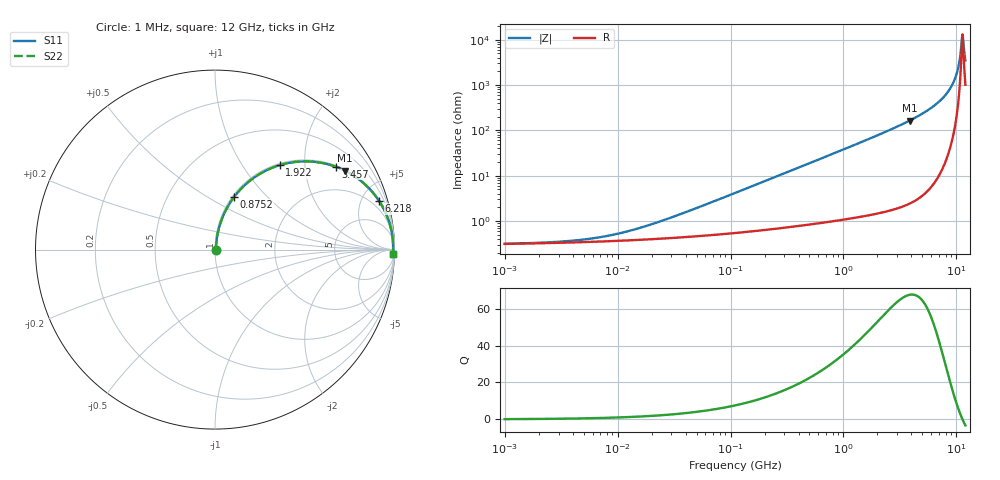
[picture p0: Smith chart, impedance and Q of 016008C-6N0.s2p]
# MHz S MA R 50
!Freq  MagS11  AngS11  MagS21  AngS21  MagS12  AngS12  MagS22  AngS22
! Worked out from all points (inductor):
!   801 points, 1 MHz to 12 GHz, reference 50 ohm
!   read as one part in series: L = 6 nH near 34.66 MHz
!   highest Q = 67.5 at 3.842 GHz (marker M1), where L = 6.78 nH
!   self-resonance near 11.18 GHz
!   S11 on the Smith chart (normalised r, x): 1 MHz: 1.01, +0.00; 875.2 MHz: 1.02, +0.66; 1.922 GHz: 1.03, +1.49; 3.457 GHz: 1.04, +2.87; 6.218 GHz: 1.13, +6.72; 12 GHz: 21, -66
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1  0.003158 6.8  0.9969 -0.0  0.9969 -0.0  0.003158 6.8
4.822396  0.003876 27.8  0.9966 -0.1  0.9966 -0.1  0.003876 27.8
10.34419  0.005348 46.4  0.9963 -0.2  0.9963 -0.2  0.005348 46.4
22.98406  0.009536 64.3  0.9959 -0.5  0.9959 -0.5  0.009536 64.3
110.8382  0.04188 80.1  0.9937 -2.4  0.9937 -2.4  0.04188 80.1
261.1649  0.09761 80.4  0.9885 -5.6  0.9885 -5.6  0.09761 80.4
528.267  0.1943 76.4  0.9727 -11.2  0.9727 -11.2  0.1943 76.4
875.2044  0.3123 70.0  0.9404 -18.2  0.9404 -18.2  0.3123 70.0
1304.592  0.442 62.4  0.8864 -26.2  0.8864 -26.2  0.442 62.4
1921.945  0.5926 52.6  0.7941 -36.3  0.7941 -36.3  0.5926 52.6
2517.778  0.7008 44.6  0.7017 -44.5  0.7017 -44.5  0.7008 44.6
3456.923  0.8152 34.5  0.567 -54.6  0.567 -54.6  0.8152 34.5
3842.205  0.8479 31.2  0.5178 -58.0  0.5178 -58.0  0.8479 31.2
6217.826  0.9535 16.5  0.2839 -72.4  0.2839 -72.4  0.9535 16.5
7863.54  0.9798 9.8  0.1709 -78.3  0.1709 -78.3  0.9798 9.8
9268.379  0.9896 5.3  0.09331 -80.9  0.09331 -80.9  0.9896 5.3
10181.12  0.9921 2.8  0.04961 -79.4  0.04961 -79.4  0.9921 2.8
10423.02  0.9924 2.2  0.03882 -77.6  0.03882 -77.6  0.9924 2.2
10924.19  0.9926 0.9  0.01789 -65.0  0.01789 -65.0  0.9926 0.9
11183.75  0.9925 0.3  0.009265 -35.4  0.009265 -35.4  0.9925 0.3
11584.69  0.992 -0.6  0.01351 53.6  0.01351 53.6  0.992 -0.6
12000  0.9913 -1.6  0.02856 71.6  0.02856 71.6  0.9913 -1.6
